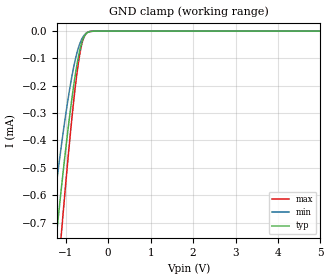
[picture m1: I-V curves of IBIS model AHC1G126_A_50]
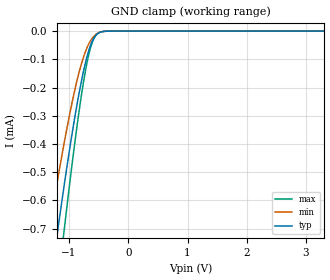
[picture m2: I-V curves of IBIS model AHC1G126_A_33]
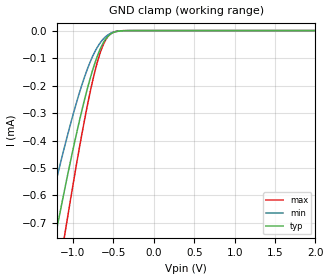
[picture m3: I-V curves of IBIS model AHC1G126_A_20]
| TEXAS INSTRUMENTS INCORPORATED
| Standard Linear and Logic Group
| IBIS Model of SN74AHC1G126
| SINGLE BUS BUFFER GATE WITH 3-STATE OUTPUT
| This file contains package information for the following:
|  SOT 5-pin (DBV) package as [Component] AHC1G126_DBV
|  SOT 5-pin (DCK) package as [Component] AHC1G126_DCK
|  SOT 5-pin (DRL) package as [Component] AHC1G126_DRL
| This device can be powered at the following Vccs:
|  5 volt Vcc
|  3.3 volt Vcc
|  2 volt Vcc
| This file provides unique models under the [Model Selector] for each Vcc.
| For operation at a specific Vcc, select the appropriate model after each
| [Model Selector] keyword.
[IBIS Ver]   3.2
[Comment char]  |_char
[File Name]   sn74ahc1g126.ibs
[File Rev]   1.1 | x_die
[Date]   August 24, 2007
[Source]   Data created from TI-SPICE simulations at TI-SLL.
[Notes]   The following is an IBIS list for the SN74AHC1G126.
   Please contact sllibis@ti.com with questions and
   comments concerning SLL IBIS models.
   - FILE REV HISTORY
   - 1.1 Release IBIS file on 09/21/07
   - C_comp values are taken at a different test condition
   than the data sheet.
   - Power clamp data was deleted in the input models as there is
   no power-clamp diode.
[Disclaimer] Property of Texas Instruments Incorporated.  Unauthorized
   reproduction and/or distribution is strictly prohibited.
   This product is protected under copyright law.
   Created  2007, (C) Copyright  2007, Texas Instruments
   Incorporated, All Rights Reserved
   UNLESS THERE IS A SIGNED, WRITTEN AGREEMENT TO THE
   CONTRARY, TEXAS INSTRUMENTS (TI) IS PROVIDING THE IBIS
   MODELS  AND WITHOUT ANY WARRANTY, EXPRESSED OR
   IMPLIED.  TI assumes no liability for:
   1) the accuracy of the IBIS models provided to your
   company;
   2) the proper functioning of these IBIS Models in your
   design or for any resulting applications; or
   3) infringement of patents, copyrights or intellectual
   property rights resulting from your use of these IBIS
   models.
   TI provides IBIS Models as a service to our customers.
   You and your company shall not distribute, sell or give
   these models to anyone else without prior written
   permission from TI.
   TI reserves the right to make changes to our products or
   to discontinue any semiconductor product or service
   without notice, and advises our customers to obtain the
   latest version of relevant information to verify, before
   placing orders, that the information being relied on is
   current.
   Please be aware that your receipt and use of the IBIS
   information provided shall serve as acceptance of these
   terms and conditions.  If you do not accept these terms,
   you should return or destroy the IBIS models and any
   other accompanying information immediately.
| Component SN74AHC1G126_DBV 5-PIN SOT
[Component]   SN74AHC1G126_DBV
[Manufacturer]   Texas Instruments, Inc.
[Package]
|   typ   min   max
R_pkg   2.500e-02   2.100e-02   2.900e-02
L_pkg   1.529e-09   1.312e-09   1.906e-09
C_pkg   1.560e-13   1.100e-13   2.400e-13
[Pin]   signal_name   model_name   R_pin   L_pin   C_pin
1   OE   AHC1G126_OE   2.100e-02   1.511e-09   1.440e-13
2   A   AHC1G126_A   2.300e-02   1.312e-09   1.380e-13
3   GND   GND   2.900e-02   1.906e-09   2.400e-13
4   Y   AHC1G126_Y   2.600e-02   1.541e-09   1.500e-13
5   VCC   POWER   2.500e-02   1.374e-09   1.100e-13
| Component SN74AHC1G126_DCK 5-PIN SOT
[Component]   SN74AHC1G126_DCK
[Manufacturer]   Texas Instruments, Inc.
[Package]
|   typ   min   max
R_pkg   2.000e-02   1.700e-02   2.500e-02
L_pkg   9.980e-10   8.810e-10   1.069e-09
C_pkg   1.460e-13   1.180e-13   2.050e-13
[Pin]   signal_name   model_name   R_pin   L_pin   C_pin
1   OE   AHC1G126_OE   1.900e-02   1.069e-09   1.620e-13
2   A   AHC1G126_A   1.800e-02   8.810e-10   1.210e-13
3   GND   GND   1.700e-02   1.031e-09   2.050e-13
4   Y   AHC1G126_Y   2.000e-02   9.600e-10   1.240e-13
5   VCC   POWER   2.500e-02   1.049e-09   1.180e-13
| Component SN74AHC1G126_DRL 5-PIN SOT
[Component]   SN74AHC1G126_DRL
[Manufacturer]   Texas Instruments, Inc.
[Package]
|   typ   min   max
R_pkg   3.200e-02   2.800e-02   3.500e-02
L_pkg   9.160e-10   7.230e-10   1.135e-09
C_pkg   2.210e-13   1.030e-13   3.740e-13
[Pin]   signal_name   model_name   R_pin   L_pin   C_pin
1   OE   AHC1G126_OE   3.400e-02   7.230e-10   1.030e-13
2   A   AHC1G126_A   2.800e-02   8.930e-10   2.370e-13
3   GND   GND   2.900e-02   1.072e-09   3.740e-13
4   Y   AHC1G126_Y   3.500e-02   7.600e-10   1.130e-13
5   VCC   POWER   3.300e-02   1.135e-09   2.800e-13
| Model AHC1G126_A
[Model Selector]   AHC1G126_A
AHC1G126_A_50   5 volt Vcc
AHC1G126_A_33   3.3 volt Vcc
AHC1G126_A_20   2 volt Vcc
| Model AHC1G126_OE
[Model Selector]   AHC1G126_OE
AHC1G126_OE_50   5 volt Vcc
AHC1G126_OE_33   3.3 volt Vcc
AHC1G126_OE_20   2 volt Vcc
| Model AHC1G126_Y
[Model Selector]   AHC1G126_Y
AHC1G126_Y_50   5 volt Vcc
AHC1G126_Y_33   3.3 volt Vcc
AHC1G126_Y_20   2 volt Vcc
| Models and submodels in the file (9): AHC1G126_A_50 (Input), AHC1G126_A_33 (Input), AHC1G126_A_20 (Input), AHC1G126_OE_50 (Input), AHC1G126_OE_33 (Input), AHC1G126_OE_20 (Input), AHC1G126_Y_50 (3-state), AHC1G126_Y_33 (3-state), AHC1G126_Y_20 (3-state)
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[Model]   AHC1G126_A_50
Model_type  Input
Vinl=1.65
Vinh=3.85
| variable   typ   min   max
C_comp   0.92pF   0.80pF   1.03pF
[Temperature Range]   40   100   -40
| Ambient temperature   25   85   -40
[Voltage range]   5   4.5   5.5
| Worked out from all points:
|   GND clamp passes 1 mA (typ) near -1.38 V on its own axis
[GND Clamp]
| AHC1G126_A_50
|   Voltage   I(typ)   I(min)   I(max)
-5V       -7.834mA   -6.491mA   -8.926mA
-1.4V     -1.031mA   -788.3uA   -1.305mA
-1.345V   -943.5uA   -717uA     -1.198mA
-1.22V    -749.9uA   -559.7uA   -959.9uA
-1.195V   -712.2uA   -529.2uA   -913uA
-1.105V   -579.3uA   -422.4uA   -746.6uA
-1.08V    -543.4uA   -393.8uA   -701.3uA
-890mV    -289.7uA   -197.1uA   -375.4uA
-725mV    -114.1uA   -74.02uA   -143.2uA
-605mV    -34.41uA   -24.51uA   -38.71uA
-475mV    -4.506uA   -3.59uA    -3.661uA
5V        7.166nA    474.1pA    66.12nA
[Model]   AHC1G126_A_33
Model_type  Input
Vinl=0.9
Vinh=2.1
| variable   typ   min   max
C_comp   0.93pF   0.82pF   1.06pF
[Temperature Range]   40   100   -40
| Ambient temperature   25   85   -40
[Voltage range]   3.3   3   3.6
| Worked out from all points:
|   GND clamp passes 1 mA (typ) near -1.38 V on its own axis
[GND Clamp]
| AHC1G126_A_33
|   Voltage   I(typ)   I(min)   I(max)
-3.3V     -4.463mA   -3.643mA   -5.247mA
-1.365V   -975.1uA   -742.8uA   -1.237mA
-1.325V   -912uA     -691.3uA   -1.16mA
-1.205V   -727.2uA   -541.3uA   -931.7uA
-1.17V    -674.8uA   -499uA     -866.3uA
-1.08V    -543.4uA   -393.8uA   -701.3uA
-885mV    -283.6uA   -192.6uA   -367.4uA
-740mV    -127.5uA   -82.68uA   -160.9uA
-625mV    -43.98uA   -30.44uA   -50.86uA
-565mV    -19.84uA   -15.07uA   -20.7uA
-505mV    -7.613uA   -6.114uA   -6.771uA
3.3V      1.837nA    303.9pA    8.84nA
[Model]   AHC1G126_A_20
Model_type  Input
Vinl=0.5
Vinh=1.5
| variable   typ   min   max
C_comp   0.92pF   0.81pF   1.01pF
[Temperature Range]   40   100   -40
| Ambient temperature   25   85   -40
[Voltage range]   2   2   2
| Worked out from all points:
|   GND clamp passes 1 mA (typ) near -1.38 V on its own axis
[GND Clamp]
| AHC1G126_A_20
|   Voltage   I(typ)   I(min)   I(max)
-2V       -2.045mA   -1.623mA   -2.511mA
-1.36V    -967.2uA   -736.3uA   -1.228mA
-1.2V     -719.7uA   -535.2uA   -922.3uA
-1.1V     -572.1uA   -416.7uA   -737.5uA
-1.075V   -536.3uA   -388.1uA   -692.3uA
-920mV    -327uA     -225.1uA   -424uA
-765mV    -151.1uA   -98.33uA   -192.3uA
-660mV    -64.49uA   -42.95uA   -77.46uA
-560mV    -18.42uA   -14.1uA    -19uA
-495mV    -6.404uA   -5.145uA   -5.513uA
-375mV    -660.8nA   -521.3nA   -330.8nA
2V        456.3pA    204.7pA    614.8pA
